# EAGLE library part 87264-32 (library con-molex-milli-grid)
RECEPTACAL
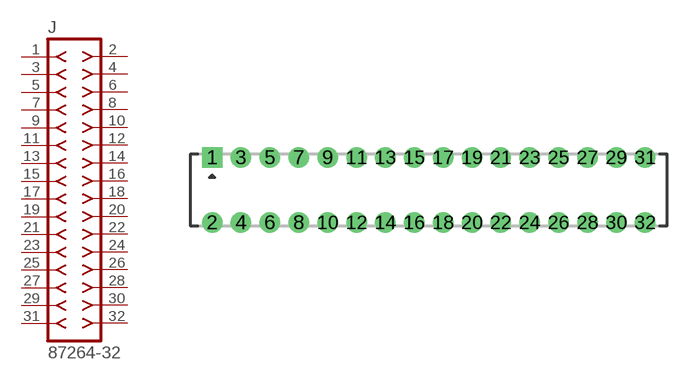
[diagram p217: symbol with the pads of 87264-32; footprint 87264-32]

Designator prefix J

## 87264-32  [87264-32]
1  1  pas
2  2  pas
3  3  pas
4  4  pas
5  5  pas
6  6  pas
7  7  pas
8  8  pas
9  9  pas
10  10  pas
11  11  pas
12  12  pas
13  13  pas
14  14  pas
15  15  pas
16  16  pas
17  17  pas
18  18  pas
19  19  pas
20  20  pas
21  21  pas
22  22  pas
23  23  pas
24  24  pas
25  25  pas
26  26  pas
27  27  pas
28  28  pas
29  29  pas
30  30  pas
31  31  pas
32  32  pas

## Footprint 87264-32 (pad centres in mm)
RECEPTACAL Dual Row, Side Entry
drill 0.914 square: 1 -15,2.25
drill 0.914: 2 -15,-2.25; 3 -13,2.25; 4 -13,-2.25; 5 -11,2.25; 6 -11,-2.25; 7 -9,2.25; 8 -9,-2.25; 9 -7,2.25; 10 -7,-2.25; 11 -5,2.25; 12 -5,-2.25; 13 -3,2.25; 14 -3,-2.25; 15 -1,2.25; 16 -1,-2.25; 17 1,2.25; 18 1,-2.25; 19 3,2.25; 20 3,-2.25; 21 5,2.25; 22 5,-2.25; 23 7,2.25; 24 7,-2.25; 25 9,2.25; 26 9,-2.25; 27 11,2.25; 28 11,-2.25; 29 13,2.25; 30 13,-2.25; 31 15,2.25; 32 15,-2.25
